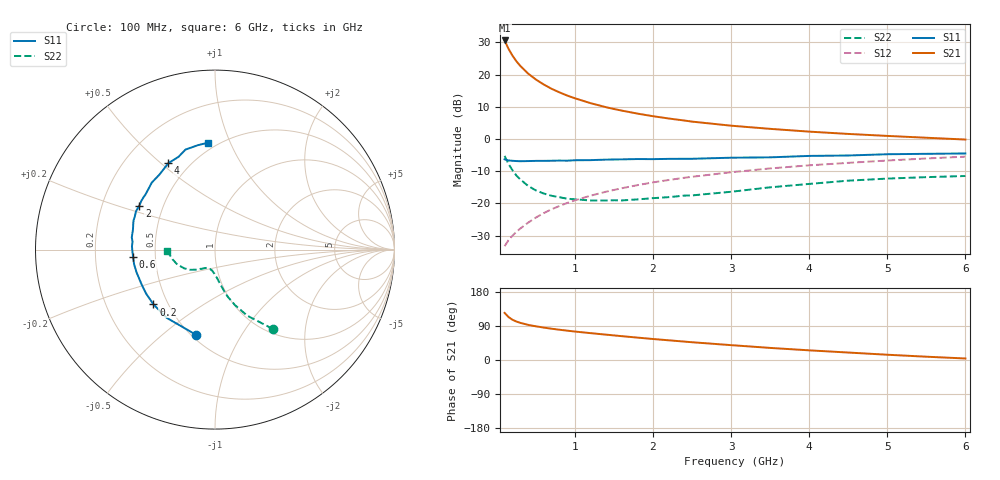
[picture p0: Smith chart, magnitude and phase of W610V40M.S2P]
! SIEMENS Small Signal Semiconductors
! BFR193W
! Si NPN RF Bipolar Junction Transistor in SOT323
! VCE = 10 V  IC = 40 mA
! Common Emitter S-Parameters:  September  1992
# GHz  S  MA  R  50
!  f  S11  S21  S12  S22
! GHz  MAG  ANG  MAG  ANG  MAG  ANG  MAG  ANG
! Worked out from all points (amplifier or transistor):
!   28 points, 100 MHz to 6 GHz, reference 50 ohm
!   highest |S21| = 30.6 dB at 100 MHz (marker M1)
!   |S21| within 3 dB of that: start of sweep to 159.7 MHz
!   unconditionally stable (mu >= 1): 647.3 MHz to 2.717 GHz
!   at 300 MHz: K = 0.86, MSG = 25.3 dB, |S12| = -27.8 dB
!   at 1.5 GHz: K = 1.03, MAG = 11.5 dB, |S12| = -15.8 dB
!   at 6 GHz: K = 0.91, MSG = 2.7 dB, |S12| = -5.5 dB
!   S11 on the Smith chart (normalised r, x): 100 MHz: 0.53, -0.65; 200 MHz: 0.42, -0.32; 600 MHz: 0.37, -0.04; 2 GHz: 0.37, +0.24; 4 GHz: 0.38, +0.53; 6 GHz: 0.45, +0.83
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0.1  0.4854 -102.9  33.98 124.3  0.0217 58.9  0.547 -53.9
0.15  0.4657 -125.2  25.21 113.3  0.0269 58.3  0.4106 -63.9
0.2  0.4591 -138.3  19.81 106.2  0.0315 59.7  0.3286 -70.2
0.25  0.4554 -147.4  16.21 101.6  0.0362 61.8  0.2721 -74.9
0.3  0.4528 -153.9  13.71 98.1  0.0407 63.8  0.2365 -77.6
0.4  0.4551 -163.7  10.42 92.8  0.0502 66.5  0.1876 -82.2
0.5  0.4582 -169.7  8.412 88.9  0.0604 68.4  0.1596 -85.7
0.6  0.4581 -174.9  7.049 85.6  0.0707 69.1  0.1427 -89.6
0.7  0.4604 -178.8  6.046 82.6  0.081 69.9  0.1316 -92.1
0.8  0.4631 177.7  5.325 79.9  0.0911 70.1  0.1251 -95.1
0.9  0.4615 174.5  4.741 77.5  0.1016 70.1  0.1184 -97.2
1  0.4686 171.7  4.299 75.1  0.1117 70.0  0.116 -99.5
1.2  0.4706 166.2  3.611 70.9  0.132 69.3  0.1111 -105.3
1.5  0.4819 160.2  2.93 64.9  0.162 67.8  0.1121 -112.0
2  0.4876 149.8  2.264 55.4  0.2122 64.5  0.1208 -120.5
2.2  0.4923 146.4  2.086 52.0  0.2312 63.1  0.1252 -122.6
3  0.5132 133.3  1.613 39.2  0.3052 56.7  0.1518 -132.6
3.5  0.5199 126.6  1.44 31.9  0.3499 52.4  0.1781 -140.8
4  0.5472 118.4  1.304 25.5  0.3908 48.1  0.201 -148.7
4.5  0.5553 111.5  1.201 19.7  0.4267 44.0  0.2259 -158.4
5.5  0.5896 99.2  1.048 8.7  0.4992 36.1  0.2561 -174.5
6  0.5972 93.6  0.983 4.0  0.533 32.0  0.2668 -178.7
